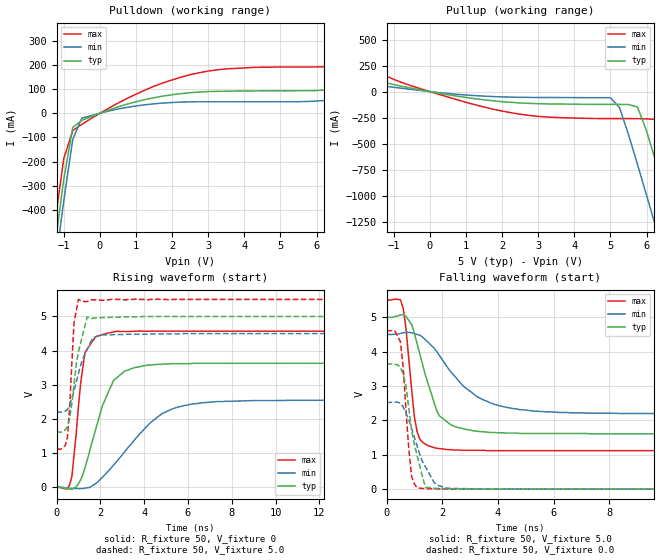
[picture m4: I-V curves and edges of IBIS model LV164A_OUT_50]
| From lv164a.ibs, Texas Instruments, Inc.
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|   Model LV164A_OUT_50
[Model]   LV164A_OUT_50
Model_type  Output
Polarity   Non-Inverting
Vmeas = 2.50v
Cref = 15pf
| variable   typ   min   max
C_comp   4.62pf   3.47pf   5.77pf
[Temperature Range]   25   85   -40
[Voltage Range]   5.0   4.5   5.5
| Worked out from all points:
|   slope of the pulldown table from 0 to 0.75 V, typ, clamps not added: 19.9 ohm
|   slope of the pullup table from 0 to 0.75 V, typ, clamps not added: 17.2 ohm
|   rising waveform, R_fixture 50, V_fixture 0: 20-80 % time 1.08ns typ, 2.17ns min, 440ps max; typ from 0 V to 3.63 V
|   falling waveform, R_fixture 50, V_fixture 5.0: 20-80 % time 731ps typ, 1.56ns min, 321ps max; typ from 5 V to 1.61 V
|   rising waveform, R_fixture 50, V_fixture 5.0: 20-80 % time 478ps typ, 677ps min, 223ps max; typ from 1.61 V to 5 V
|   falling waveform, R_fixture 50, V_fixture 0.0: 20-80 % time 464ps typ, 703ps min, 253ps max; typ from 3.64 V to 0 V
[Pulldown]
|   Voltage   I(typ)   I(min)   I(max)
-5V       -5.14A     -5.22A     -5.05A
-1.25V    -557mA     -649mA     -461mA
-1V       -274mA     -363mA     -188mA
-750mV    -58.9mA    -108mA     -71.3mA
-500mV    -29.2mA    -20mA      -46.2mA
0V        -3.33nA    -3.4nA     -3.57nA
1.25V     56.7mA     35.2mA     96mA
2.5V      85.3mA     47.3mA     160mA
3.5V      91.4mA     47.8mA     184mA
7V        108mA      63mA       206mA
8.25V     142mA      85.5mA     255mA
10V       202mA      122mA      357mA
[Pullup]
|   Voltage   I(typ)   I(min)   I(max)
-5V       328mA      183mA      611mA
-3.75V    271mA      154mA      499mA
1.5V      -78.8mA    -43.5mA    -148mA
3V        -116mA     -56.1mA    -238mA
5V        -123mA     -58.9mA    -259mA
5.25V     -123mA     -153mA     -259mA
5.75V     -147mA     -699mA     -260mA
6.25V     -664mA     -1.29A     -268mA
6.5V      -960mA     -1.6A      -403mA
6.75V     -1.26A     -1.9A      -685mA
7.25V     -1.87A     -2.51A     -1.28A
10V       -5.25A     -5.89A     -4.66A
[Ramp]
| variable   typ   min   max
dV/dt_r   2.18E+00/1.05E-09   1.54E+00/2.16E-09   2.74E+00/4.28E-10
dV/dt_f   2.08E+00/7.60E-10   1.41E+00/1.58E-09   2.66E+00/3.79E-10
R_load = 50
[Rising Waveform]
R_fixture = 50
V_fixture = 0
|   Time   V(typ)   V(min)   V(max)
0s        0V         0V         0V
500ps     -40.3mV    -21.2mV    -36.1mV
700ps     -52.7mV    -31.1mV    316mV
1.1ns     219mV      -37.1mV    3.04V
1.3ns     580mV      -23.5mV    3.95V
2.3ns     2.69V      432mV      4.51V
3.1ns     3.4V       1.03V      4.56V
4.8ns     3.6V       2.15V      4.57V
6.3ns     3.63V      2.45V      4.57V
25ns      3.63V      2.55V      4.57V
[Falling Waveform]
R_fixture = 50
V_fixture = 5.0
V_fixture_min = 4.5
V_fixture_max = 5.5
|   Time   V(typ)   V(min)   V(max)
0s        5V         4.5V       5.5V
500ps     5.07V      4.53V      5.51V
700ps     5.03V      4.56V      4.67V
1ns       4.54V      4.52V      2.11V
1.1ns     4.23V      4.5V       1.67V
1.8ns     2.29V      4.01V      1.19V
2.3ns     1.88V      3.42V      1.15V
3.3ns     1.68V      2.67V      1.13V
5.3ns     1.62V      2.27V      1.12V
25ns      1.61V      2.2V       1.12V
[Rising Waveform]
R_fixture = 50
V_fixture = 5.0
V_fixture_min = 4.5
V_fixture_max = 5.5
|   Time   V(typ)   V(min)   V(max)
0s        1.61V      2.2V       1.12V
400ps     1.68V      2.23V      1.23V
500ps     1.78V      2.28V      1.47V
600ps     2.03V      2.41V      2.35V
800ps     3.02V      2.83V      4.83V
1ns       3.97V      3.33V      5.5V
1.4ns     4.99V      4.04V      5.44V
1.7ns     4.95V      4.39V      5.49V
2.1ns     4.97V      4.47V      5.47V
25ns      5V         4.5V       5.5V
[Falling Waveform]
R_fixture = 50
V_fixture = 0.0
|   Time   V(typ)   V(min)   V(max)
0s        3.64V      2.53V      4.61V
500ps     3.54V      2.5V       4.29V
600ps     3.35V      2.39V      3.52V
700ps     3V         2.22V      2.27V
900ps     1.72V      1.77V      371mV
1.1ns     978mV      1.25V      30.8mV
1.4ns     47.8mV     645mV      15.8mV
1.8ns     21.7mV     124mV      7.66mV
2.2ns     12.6mV     24.3mV     4.01mV
25ns      0V         0V         7.74uV
